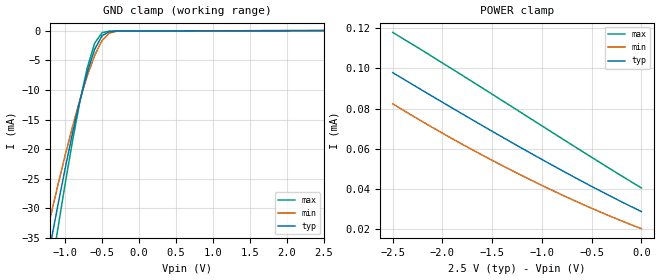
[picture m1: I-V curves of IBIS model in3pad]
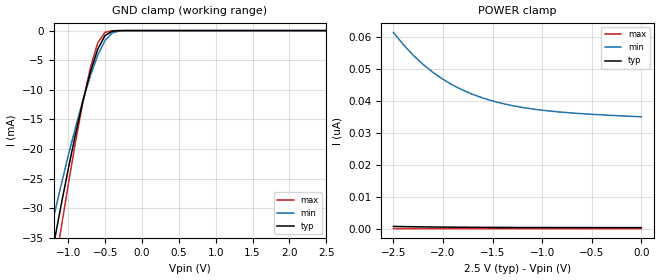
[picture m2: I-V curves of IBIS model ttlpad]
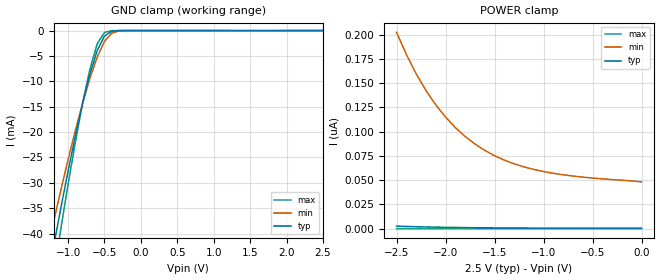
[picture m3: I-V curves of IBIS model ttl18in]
| IBIS file idt45t915z.ibs created by s2ibis2 version 1.2
| North Carolina State University Electronics Research Laboratory  1995
[IBIS ver]   3.2
[File name]   idt45t915z.ibs
[File Rev]   1.0
[Date]   Friday, November 09, 2001
[Source]   Integrated Device Technology, Inc.
[Notes]   Input pins <A> and <AX> can be configured as one of the
   following three models: ttl25in, ttl18in, or hstlin.
   Output pins <Q1> to <Q5X> can be configured as one of the
   following three models: ttl25out, ttl18out, or hstlout.
   Please change the column 'model_name' in pin list to select
   the correct model.
[Disclaimer] Integrated Device Technology, Inc. ("IDT") hereby grants the
   user of this IBIS model a non-exclusive, nontransferable
   license to use this IBIS model under the following terms. The
   user is granted this license only to use the IBIS model and is
   not granted rights to sell, copy (except as needed to run the
   IBIS model), rent, lease or sub-license the IBIS model in
   whole or in part, or in modified form to anyone. The User may
   modify the IBIS model to suit its specific applications, but
   rights to derivative works and such modifications shall belong
   to IDT. This IBIS model is provided on an AS IS" basis and IDT
   makes absolutely no warranty with respect to the information
   contained herein. IDT DISCLAIMS AND CUSTOMER WAIVES ALL
   WARRANTIES, EXPRESS AND IMPLIED, INCLUDING WARRANTIES OF
   MERCHANTABILITY AND FITNESS FOR A PARTICULAR PURPOSE. THE
   ENTIRE RISK AS TO QUALITY AND PERFORMANCE IS WITH THE USER
   ACCORDINGLY, IN NO EVENT SHALL IDT BE LIABLE FOR ANY DIRECT OR
   INDIRECT DAMAGES, WHETHER IN CONTRACT OR TORT, INCLUDING ANY
   LOST PROFITS OR OTHER INCIDENTAL, CONSEQUENTIAL, EXEMPLARY, OR
   PUNITIVE DAMAGES ARISING OUT OF THE USE OR APPLICATION OF THE
   IBIS model. Further, IDT reserves the right to make changes
   without notice to any product herein to improve reliability,
   function, or design. IDT does not convey any license under
   patent rights or any other intellectual property rights,
   including those of third parties. IDT is not obligated to
   provide maintenance or support for the licensed IBIS model.
[Copyright]   Copyright 2001, Integrated Device Technology, Inc. all rights
   reserved
|   Component idt45t915z
[Component]   idt45t915z
[Manufacturer]   Integrated Device Technology
|Package   PA48
[Package]
| variable   typ   min   max
R_pkg   6.00000m   6.00000m   6.00000m
L_pkg   3.00000nH   3.00000nH   3.00000nH
C_pkg   0.20000pF   0.20000pF   0.20000pF
[Pin]  signal_name   model_name   R_pin   L_pin   C_pin
1   GL   ttlpad
2   VDD   POWER
3   VDD   POWER
4   GND   GND
5   GND   GND
6   GPX   ttlpad
7   VDDQ   POWER
8   Q1X   ttl25out
9   Q1   ttl25out
10   GND   GND
11   VDDQ   POWER
12   AX   ttl25in
13   A   ttl25in
14   VDDQ   POWER
15   GND   GND
16   Q5X   ttl25out
17   Q5   ttl25out
18   VDDQ   POWER
19   GMX   ttlpad
20   GND   GND
21   GND   GND
22   VDD   POWER
23   VDD   POWER
24   RxS   in3pad
25   TxS   in3pad
26   GND   GND
27   VDDQ   POWER
28   GND   GND
29   GND   GND
30   VDDQ   POWER
31   VDDQ   POWER
32   Q4   ttl25out
33   Q4X   ttl25out
34   GND   GND
35   VDDQ   POWER
36   Q3   ttl25out
37   Q3X   ttl25out
38   VDDQ   POWER
39   GND   GND
40   Q2   ttl25out
41   Q2X   ttl25out
42   VDDQ   POWER
43   GND   GND
44   GND   GND
45   GND   GND
46   VDDQ   POWER
47   VDDQ   POWER
48   GND   GND
[Pin Mapping]  pulldown_ref   pullup_ref   gnd_clamp_ref   power_clamp_ref
1   gnd   vdd
2   NC   vdd
3   NC   vdd
4   gnd   NC
5   gnd   NC
6   gnd   vdd
7   NC   vddq
8   gnd   vddq
9   gnd   vddq
10   gnd   NC
11   NC   vddq
12   gnd   vdd
13   gnd   vdd
14   NC   vddq
15   gnd   NC
16   gnd   vddq
17   gnd   vddq
18   NC   vddq
19   gnd   vdd
20   gnd   NC
21   gnd   NC
22   NC   vdd
23   NC   vdd
24   gnd   vdd
25   gnd   vdd
26   gnd   NC
27   NC   vddq
28   gnd   NC
29   gnd   NC
30   NC   vddq
31   NC   vddq
32   gnd   vddq
33   gnd   vddq
34   gnd   NC
35   NC   vddq
36   gnd   vddq
37   gnd   vddq
38   NC   vddq
39   gnd   NC
40   gnd   vddq
41   gnd   vddq
42   NC   vddq
43   gnd   NC
44   gnd   NC
45   gnd   NC
46   NC   vddq
47   NC   vddq
48   gnd   NC
| Models and submodels in the file (8): in3pad (Input), ttlpad (Input), ttl18in (Input), ttl25in (Input), hstlin (Input), ttl18out (Output), ttl25out (Output), hstlout (Output)
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|   Model in3pad
[Model]   in3pad
Model_type   Input
Polarity   Non-Inverting
Vinl =  0.70000V
Vinh =  1.70000V
Vmeas =  1.25000V
C_comp   5.00000pF   5.00000pF   5.00000pF
[Temperature Range]   45.00000   0.14000k   -30.00000
[Voltage Range]   2.50000V   2.30000V   2.70000V
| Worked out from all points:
|   GND clamp passes 1 mA (typ) near -0.51 V on its own axis
[GND_clamp]
| voltage   I(typ)   I(min)   I(max)
-2.5V     -129.2mA   -109.1mA   -150.7mA
-1.3V     -43.03mA   -37.1mA    -49.76mA
-1.2V     -36.26mA   -31.58mA   -41.61mA
-1.1V     -29.68mA   -26.24mA   -33.65mA
-900mV    -17.38mA   -16.25mA   -18.7mA
-800mV    -11.87mA   -11.72mA   -12.03mA
-700mV    -7.017mA   -7.631mA   -6.282mA
-600mV    -3.163mA   -4.169mA   -2.108mA
-500mV    -846.7uA   -1.655mA   -328.1uA
-400mV    -132.2uA   -398uA     -66.99uA
-300mV    -41.75uA   -74.33uA   -49.92uA
2.5V      28.85uA    24.24uA    34.77uA
[POWER_clamp]
| voltage   I(typ)   I(min)   I(max)
-2.5V     97.81uA    82.34uA    117.8uA
-1.9V     80.2uA     64.99uA    99.56uA
-1.5V     68.7uA     54.27uA    87.12uA
-1.2V     60.25uA    46.68uA    77.7uA
-600mV    43.96uA    32.66uA    58.9uA
-300mV    36.22uA    26.27uA    49.65uA
0V        28.85uA    20.35uA    40.61uA
|   Model ttlpad
[Model]   ttlpad
Model_type   Input
Polarity   Non-Inverting
Vinl =  0.70000V
Vinh =  1.70000V
Vmeas =  1.25000V
C_comp   5.00000pF   5.00000pF   5.00000pF
[Temperature Range]   45.00000   0.14000k   -30.00000
[Voltage Range]   2.50000V   2.30000V   2.70000V
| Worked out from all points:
|   GND clamp passes 1 mA (typ) near -0.51 V on its own axis
[GND_clamp]
| voltage   I(typ)   I(min)   I(max)
-2.5V     -129.2mA   -109.1mA   -150.6mA
-1.3V     -43.01mA   -37.08mA   -49.74mA
-1.2V     -36.24mA   -31.57mA   -41.59mA
-1.1V     -29.66mA   -26.23mA   -33.63mA
-900mV    -17.36mA   -16.23mA   -18.68mA
-800mV    -11.85mA   -11.7mA    -12mA
-700mV    -6.996mA   -7.615mA   -6.253mA
-600mV    -3.137mA   -4.151mA   -2.071mA
-500mV    -815.1uA   -1.634mA   -278.8uA
-400mV    -95.37uA   -373.7uA   -14.75uA
-300mV    -5.658uA   -48.78uA   -281.7nA
2.5V      324.7pA    35.28nA    828.2fA
[POWER_clamp]
| voltage   I(typ)   I(min)   I(max)
-2.5V     698.6pA    61.39nA    2.05pA
-2.4V     644.6pA    57.56nA    1.88pA
-2.3V     597.5pA    54.23nA    1.737pA
-2.2V     556.7pA    51.34nA    1.611pA
-2.1V     521.4pA    48.85nA    1.499pA
-1.9V     465pA      44.88nA    1.333pA
-1.8V     442.7pA    43.32nA    1.256pA
-1.6V     407.7pA    40.88nA    1.155pA
-1.3V     373.1pA    38.48nA    1.037pA
-1V       352.5pA    37.05nA    965.9fA
-600mV    337.2pA    35.97nA    899.5fA
0V        324.7pA    34.99nA    849.9fA
|   Model ttl18in
[Model]   ttl18in
Model_type   Input
Polarity   Non-Inverting
Vinl =  0.68V
Vinh =  1.07V
Vmeas =  0.9V
C_comp   5.00000pF   5.00000pF   5.00000pF
[Temperature Range]   45.00000   0.14000k   -30.00000
[Voltage Range]   2.50000V   2.30000V   2.70000V
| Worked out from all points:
|   GND clamp passes 1 mA (typ) near -0.49 V on its own axis
[GND_clamp]
| voltage   I(typ)   I(min)   I(max)
-2.5V     -150.1mA   -128.5mA   -173mA
-1.3V     -50.47mA   -44.23mA   -57.51mA
-1.2V     -42.64mA   -37.76mA   -48.2mA
-1.1V     -35.02mA   -31.48mA   -39.1mA
-900mV    -20.73mA   -19.68mA   -21.96mA
-800mV    -14.28mA   -14.3mA    -14.26mA
-700mV    -8.553mA   -9.407mA   -7.567mA
-600mV    -3.939mA   -5.223mA   -2.609mA
-500mV    -1.074mA   -2.122mA   -375.8uA
-400mV    -131.3uA   -507.1uA   -20.31uA
-300mV    -7.825uA   -67.79uA   -384.6nA
2.5V      443.6pA    49.9nA     1.135pA
[POWER_clamp]
| voltage   I(typ)   I(min)   I(max)
-2.5V     2.616nA    202.4nA    8.153pA
-2.4V     2.294nA    179.5nA    7.17pA
-2.3V     2.014nA    159.7nA    6.305pA
-2.2V     1.772nA    142.5nA    5.573pA
-2.1V     1.564nA    127.7nA    4.925pA
-1.9V     1.231nA    104.2nA    3.911pA
-1.8V     1.1nA      95.05nA    3.496pA
-1.6V     895.6pA    80.73nA    2.854pA
-1.3V     696.3pA    66.86nA    2.22pA
-1V       581.4pA    58.89nA    1.825pA
-600mV    500.6pA    53.16nA    1.519pA
0V        443.6pA    48.28nA    1.265pA
